DATA_BLOCK DB 5
TITLE =BLOCK DATA FOR REAL VALUE
AUTHOR : Esposito
FAMILY : EGAL_srl
NAME : DB_REAL
VERSION : 0.1


  STRUCT
   MIS0 : ARRAY  [0 .. 100 ] OF //DOUBLE WORD FOR ANALOGICAL VALUE
   REAL ;
  END_STRUCT ;
BEGIN
   MIS0[0] := 0.000000e+000;
   MIS0[1] := 0.000000e+000;
   MIS0[2] := 0.000000e+000;
   MIS0[3] := 0.000000e+000;
   MIS0[4] := 0.000000e+000;
   MIS0[5] := 2.600000e+000;
   MIS0[6] := 0.000000e+000;
   MIS0[7] := 1.500000e+003;
   MIS0[8] := 0.000000e+000;
   MIS0[9] := 0.000000e+000;
   MIS0[10] := 0.000000e+000;
   MIS0[11] := 1.500000e+001;
   MIS0[12] := 0.000000e+000;
   MIS0[13] := 0.000000e+000;
   MIS0[14] := 0.000000e+000;
   MIS0[15] := 0.000000e+000;
   MIS0[16] := 0.000000e+000;
   MIS0[17] := 0.000000e+000;
   MIS0[18] := 3.740000e+000;
   MIS0[19] := 0.000000e+000;
   MIS0[20] := 0.000000e+000;
   MIS0[21] := 0.000000e+000;
   MIS0[22] := 0.000000e+000;
   MIS0[23] := 0.000000e+000;
   MIS0[24] := 0.000000e+000;
   MIS0[25] := 0.000000e+000;
   MIS0[26] := 0.000000e+000;
   MIS0[27] := 0.000000e+000;
   MIS0[28] := 0.000000e+000;
   MIS0[29] := 0.000000e+000;
   MIS0[30] := 0.000000e+000;
   MIS0[31] := 0.000000e+000;
   MIS0[32] := 0.000000e+000;
   MIS0[33] := 0.000000e+000;
   MIS0[34] := 0.000000e+000;
   MIS0[35] := 0.000000e+000;
   MIS0[36] := 0.000000e+000;
   MIS0[37] := 0.000000e+000;
   MIS0[38] := 0.000000e+000;
   MIS0[39] := 0.000000e+000;
   MIS0[40] := 0.000000e+000;
   MIS0[41] := 0.000000e+000;
   MIS0[42] := 0.000000e+000;
   MIS0[43] := 0.000000e+000;
   MIS0[44] := 0.000000e+000;
   MIS0[45] := 0.000000e+000;
   MIS0[46] := 0.000000e+000;
   MIS0[47] := 0.000000e+000;
   MIS0[48] := 0.000000e+000;
   MIS0[49] := 0.000000e+000;
   MIS0[50] := 0.000000e+000;
   MIS0[51] := 0.000000e+000;
   MIS0[52] := 0.000000e+000;
   MIS0[53] := 0.000000e+000;
   MIS0[54] := 0.000000e+000;
   MIS0[55] := 0.000000e+000;
   MIS0[56] := 0.000000e+000;
   MIS0[57] := 0.000000e+000;
   MIS0[58] := 0.000000e+000;
   MIS0[59] := 0.000000e+000;
   MIS0[60] := 0.000000e+000;
   MIS0[61] := 0.000000e+000;
   MIS0[62] := 0.000000e+000;
   MIS0[63] := 0.000000e+000;
   MIS0[64] := 0.000000e+000;
   MIS0[65] := 0.000000e+000;
   MIS0[66] := 0.000000e+000;
   MIS0[67] := 0.000000e+000;
   MIS0[68] := 0.000000e+000;
   MIS0[69] := 0.000000e+000;
   MIS0[70] := 0.000000e+000;
   MIS0[71] := 0.000000e+000;
   MIS0[72] := 0.000000e+000;
   MIS0[73] := 0.000000e+000;
   MIS0[74] := 0.000000e+000;
   MIS0[75] := 0.000000e+000;
   MIS0[76] := 0.000000e+000;
   MIS0[77] := 0.000000e+000;
   MIS0[78] := 0.000000e+000;
   MIS0[79] := 0.000000e+000;
   MIS0[80] := 0.000000e+000;
   MIS0[81] := 0.000000e+000;
   MIS0[82] := 0.000000e+000;
   MIS0[83] := 0.000000e+000;
   MIS0[84] := 0.000000e+000;
   MIS0[85] := 0.000000e+000;
   MIS0[86] := 0.000000e+000;
   MIS0[87] := 0.000000e+000;
   MIS0[88] := 0.000000e+000;
   MIS0[89] := 0.000000e+000;
   MIS0[90] := 0.000000e+000;
   MIS0[91] := 0.000000e+000;
   MIS0[92] := 0.000000e+000;
   MIS0[93] := 0.000000e+000;
   MIS0[94] := 0.000000e+000;
   MIS0[95] := 0.000000e+000;
   MIS0[96] := 0.000000e+000;
   MIS0[97] := 0.000000e+000;
   MIS0[98] := 0.000000e+000;
   MIS0[99] := 0.000000e+000;
   MIS0[100] := 0.000000e+000;
END_DATA_BLOCK

